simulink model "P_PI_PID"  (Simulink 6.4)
settings: Solver=ode45  StartTime=0.0  StopTime=10.0  RelTol=1e-3
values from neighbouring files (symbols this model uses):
  Ko = tf(k, [T^3 3*T^2 3*T 1])    [zkrypt.m]
undefined symbols (not defined in the file or in its folder): kp, magnitude, s, Td, Ti

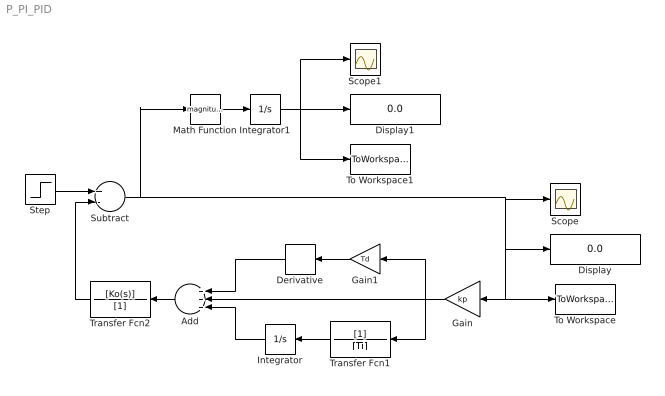
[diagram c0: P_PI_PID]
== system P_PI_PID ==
  Add : Sum  Orientation=left  Inputs=+++  OutScaling=2^-10
  Derivative : Derivative  Orientation=left
  Display : Display
  Display1 : Display
  Gain : Gain  Orientation=left  Gain=kp
  Gain1 : Gain  Orientation=left  Gain=Td
  Integrator : Integrator  Orientation=left
  Integrator1 : Integrator
  Math Function : Math  Operator=magnitude^2
  Scope : Scope
  Scope1 : Scope
  Step : Step  Time=0  SampleTime=0
  Subtract : Sum  Inputs=+-  OutScaling=2^-10
  To Workspace : ToWorkspace  VariableName=resp  SampleTime=-1  SaveFormat=Structure
  To Workspace1 : ToWorkspace  VariableName=resp1  SampleTime=-1  SaveFormat=Structure
  Transfer Fcn1 : TransferFcn  Orientation=left  Denominator=[Ti]
  Transfer Fcn2 : TransferFcn  Orientation=left  Numerator=[Ko(s)]  Denominator=[1]
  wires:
  Step/1 -> Subtract/1
  Gain/1 -> Gain1/1, Transfer Fcn1/1, Add/2
  Gain1/1 -> Derivative/1
  Derivative/1 -> Add/1
  Transfer Fcn1/1 -> Integrator/1
  Integrator/1 -> Add/3
  Subtract/1 -> Scope/1, Display/1, Gain/1, To Workspace/1, Math Function/1
  Math Function/1 -> Integrator1/1
  Integrator1/1 -> Display1/1, Scope1/1, To Workspace1/1
  Add/1 -> Transfer Fcn2/1
  Transfer Fcn2/1 -> Subtract/2
